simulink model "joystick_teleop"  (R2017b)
settings: Solver=FixedStepDiscrete  StartTime=0.0  StopTime=Inf  FixedStep=0.001  RelTol=1e-3  EnableMultiTasking=on
PostLoadFcn:
  | , if any(exist('dsrtsu_mdlpostloadfcn', 'file') == [2, 3, 6]), try dsrtsu_mdlpostloadfcn('Execute', bdroot); catch fprintf('Error in PostLoadFcn (dsrtsu_mdlpostloadfcn) for model "%s":\n %s\n', bdroot, lasterr); end, end,
libraries: vehicle_data_blocks x9, dbw_interface_blocks x5, adas_kit_info_blocks x2, simulink x2, rtican x1, vehicle_control_blocks x1

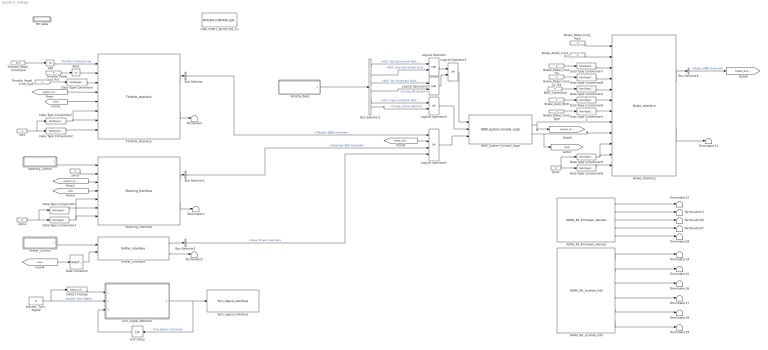
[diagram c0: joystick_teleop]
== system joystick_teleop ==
  ADAS_Kit_Firmware_Version : adas_kit_info_blocks/ADAS_Kit_Firmware_Version
  ADAS_Kit_License_Info : adas_kit_info_blocks/ADAS_Kit_License_Info
  Abs : Abs
  Abs1 : Abs
  BOO_Command : Constant  Value=0
  Brake_Auto_BOO : Constant
  Brake_Interface : dbw_interface_blocks/Brake_Interface
  Brake_Pedal_Cmd_CL_Trq : Constant  Value=0
  Brake_Pedal_Cmd_Pct : Constant  Value=0
  Brake_Pedal_Cmd_Raw : Constant  Value=0
  Brake_Pedal_Cmd_Trq : Constant  Value=0
  Brake_Pedal_Cmd_Type : Constant  Value=3
  Bus Selector : BusSelector  OutputSignals=Throttle_DBW_Override
  Bus Selector1 : BusSelector  OutputSignals=Steering_DBW_Override
  Bus Selector2 : BusSelector  OutputSignals=Gear_Driver_Override
  Bus Selector3 : BusSelector  OutputSignals=ACC_Set_Decrement_Button,ACC_Gap_Decrement_Button,ACC_Set_Increment_Button,Cruise_Off_Button,ACC_Gap_Increment_Button,Cruise_Cancel_Button
  Bus Selector4 : BusSelector  OutputSignals=Brake_DBW_Override
  CAN_TYPE1_SETUP_M1_C1 : rtican/RTICAN CONTROLLER SETUP   Reserved1=[]  Reserved2=[]  Reserved3=[]  Reserved4=[]  AcceptanceMask=[]  ArbitrationField=[]  Parameters=[]  SFcnRTICANSettings=[]  MS_Struct=[]  BoardTypeNo=[]  BoardNo=[]  ChannelNo=[]  DialogFcn=[]  UnitName=[]  Revision=[]  UnitValues=[]  DSProperties=struct('RTI',struct('Version',uint32(12),'BlockType',struct('isSLSource',uint8(0),'isSLSink',uint8(0),'isHWSource',uint8(0),'isHWSink',uint8(0),'isSetup',uint8(1),'isInline',uint8(1),'isNonInline',uint8(0),'isInterrupt',uint8(0),'isChannelwise',uint8(0)),'IOBoardType','RTICAN','UnitType','NON_MESSAGE','Identifier','MASTER','DialogType','ML','BlockSet','RTICAN','SlaveProcessor','CAN'))  RTIBlockInterface=struct('InputPortsWidth',int32(0),'InputPortsActive',0,'OutputPortsWidth',int32(0),'OutputPortsActive',0,'DialogFcn','rtican_master_setup_gui','BlockDisplay',{{['CAN CONTROLLER\n SETUP'],'center'}},'IconTransparency','on','InitLevel',3,'IWork',{{{'',uint32(2)}}},'BlockName',struct('Token',{{'CAN_TYPE','_SETUP_M','_C'}},'BlockParam',{{'BoardTypeNo','BoardNo','ChannelNo'}}),'ParameterTunableNames',{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  RTIBlockParameters=struct('BoardTypeNo',{{1,'OFF',[]}},'BoardNo',{{1,'ON',[1 16]}},'ChannelNo',{{1,'ON',[1 2]}},'AcceptanceMask',{{0,'OFF',[]}},'ArbitrationField',{{0,'OFF',[]}},'Parameters',{{struct('Config',struct('Baudrate',500,'SampleMode',1,'UsedParamSet',1,'validSettings',1,'isBTRvalues',0,'Advanced',struct('Baudrate',{500,500,500},'Frequency',{24000000,36000000,64000000},'Settings',{struct('SMPL',0,'BRP',0,'N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  RTISFcnParameters=struct('SFcnRTICANSettings','struct','SFcnRTICCPSettings','struct','SFcnRTIXCPSettings','struct','AcceptanceMask','int32','ArbitrationField','int32','TLCFileName','char')  RTIBlockParaDefault=struct('BoardTypeNo',4302,'BoardNo',1,'ChannelNo',1,'AcceptanceMask',0,'ArbitrationField',0,'Parameters',struct('Config',struct('Baudrate',500,'SampleMode',1,'UsedParamSet',1,'validSettings',1,'isBTRvalues',0,'Advanced',struct('Frequency',16000000,'BTR0',64,'BTR1',28,'Settings',struct('SMPL',0,'BRP',0,'NBT',16,'TSEG1',12,'TSEG2',1,'SJW',1,'SP',87))),'configType',1,'Options',struct('DataFileSelecte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
  DBW_System_Enable_Logic : vehicle_control_blocks/DBW_System_Enable_Logic
  Data Type Conversion{,2,4,6,11} (5 alike) : DataTypeConversion  OutDataTypeStr=uint8
  Data Type Conversion{1,3,5,9..10} (5 alike) : DataTypeConversion  OutDataTypeStr=boolean
  Data Type Conversion7 : DataTypeConversion  OutDataTypeStr=uint16
  Data Type Conversion8 : DataTypeConversion  OutDataTypeStr=uint16
  Detect Change : simulink/Logic and Bit Operations/Detect Change  vinit=0  OutDataTypeStr=boolean
  Joystick_Turn_Signal : Constant  Value=0
  Logical Operator : Logic  AllPortsSameDT=off  OutDataTypeStr=boolean
  Logical Operator1 : Logic  Operator=OR  Inputs=4  AllPortsSameDT=off  OutDataTypeStr=boolean
  Logical Operator2 : Logic  AllPortsSameDT=off  OutDataTypeStr=boolean
  Logical Operator3 : Logic  Operator=OR  AllPortsSameDT=off  OutDataTypeStr=boolean
  Logical Operator4 : Logic  Operator=OR  AllPortsSameDT=off  OutDataTypeStr=boolean
  RTI Data : Subsystem  Tag=struct('RTIDataServer',struct('RTIDataServerVs','2','RTIModelDescription','struct(''main'',''joystick_teleop'',''sub'','''',''isMp'',0)'))  LoadFcn="if exist('rtidc'), try,  rtidc('DataHostBlockClbLoad', gcbh); catch, disp(['Warning: ''LoadFcn'' for RTI Data block failed: ' lasterr]); end, end,"  mask(RTI_DATA_HOST){}
      mask help: RTI Data Block. This block is used by RTI to store internal model-dependent data. Please keep this block on the root level of the model. Deleting this block will result in data loss. NEVER DELETE OR COPY THIS BLOCK!
  Rate Transition : RateTransition
  Shifter_Control : Subsystem
  Shifter_Interface : dbw_interface_blocks/Shifter_Interface
  Steering_Control : Subsystem
  Steering_Interface : dbw_interface_blocks/Steering_Interface
  Terminator{,1..2,11..19,26..28} (15 alike) : Terminator
  Throttle_Interface : dbw_interface_blocks/Throttle_Interface
  Throttle_Pedal_Cmd_Pct : Constant  Value=0
  Throttle_Pedal_Cmd_Type : Constant  Value=2
  Throttle_Pedal_Command : Constant  Value=0.15
  Turn_Signal_Behavior : MATLAB Function  TreatAsAtomicUnit=on
  Turn_Signal_Interface : dbw_interface_blocks/Turn_Signal_Interface
  Unit Delay : UnitDelay  SampleTime=-1
  Vehicle_Data : Subsystem
  zero{,1..3} (4 alike) : Constant  Value=0
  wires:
  Throttle_Pedal_Command/1 -> Abs/1
  Abs/1 -> Throttle_Interface/1  "Throttle_Command_Sig"
  [system_enable] -> Throttle_Interface/4
  Throttle_Interface/1 -> Bus Selector/1
  Bus Selector/1 -> Logical Operator1/1  "<Throttle_DBW_Override>"
  Steering_Control/1(Steering_Command) -> Steering_Interface/1
  [system_enable] -> Steering_Interface/3
  Steering_Interface/1 -> Bus Selector1/1
  Bus Selector1/1 -> Logical Operator1/3  "<Steering_DBW_Override>"
  Steering_Interface/2 -> Terminator1/1
  Shifter_Control/1(Gear_Command) -> Shifter_Interface/1
  [clear] -> Rate Transition/1
  Rate Transition/1 -> Shifter_Interface/2
  Bus Selector2/1 -> Logical Operator1/4  "<Gear_Driver_Override>"
  Shifter_Interface/1 -> Bus Selector2/1
  Shifter_Interface/2 -> Terminator2/1
  Joystick_Turn_Signal/1 -> Detect Change/1, Turn_Signal_Behavior/2(u)  "Joystick_Turn_Signal"
  Detect Change/1 -> Turn_Signal_Behavior/1(new_u)
  Turn_Signal_Behavior/1(y) -> Turn_Signal_Interface/1, Unit Delay/1  "Turn_Signal_Command"
  Unit Delay/1 -> Turn_Signal_Behavior/3(last_y)
  Vehicle_Data/1(Misc_Report_Bus) -> Bus Selector3/1
  Bus Selector3/1 -> Logical Operator/1  "<ACC_Set_Decrement_Button>"
  Bus Selector3/2 -> Logical Operator/2  "<ACC_Gap_Decrement_Button>"
  Bus Selector3/5 -> Logical Operator4/1  "<ACC_Gap_Increment_Button>"
  [brake_override] -> Logical Operator1/2
  Logical Operator1/1 -> DBW_System_Enable_Logic/3
  DBW_System_Enable_Logic/2 -> [clear], Brake_Interface/9
  Brake_Pedal_Cmd_Raw/1 -> Brake_Interface/1
  Bus Selector4/1 -> [brake_override]  "<Brake_DBW_Override>"
  Bus Selector3/3 -> Logical Operator2/1  "<ACC_Set_Increment_Button>"
  Bus Selector3/4 -> Logical Operator2/2  "<Cruise_Off_Button>"
  Bus Selector3/6 -> Logical Operator4/2  "<Cruise_Cancel_Button>"
  Logical Operator/1 -> Logical Operator3/1
  Logical Operator2/1 -> Logical Operator3/2
  Logical Operator3/1 -> DBW_System_Enable_Logic/1
  Logical Operator4/1 -> DBW_System_Enable_Logic/2
  DBW_System_Enable_Logic/1 -> [system_enable], Brake_Interface/8
  Throttle_Interface/2 -> Terminator/1
  Brake_Interface/2 -> Terminator11/1
  Brake_Interface/1 -> Bus Selector4/1
  ADAS_Kit_License_Info/1 -> Terminator14/1
  ADAS_Kit_License_Info/2 -> Terminator15/1
  ADAS_Kit_License_Info/3 -> Terminator16/1
  ADAS_Kit_License_Info/4 -> Terminator17/1
  ADAS_Kit_License_Info/5 -> Terminator18/1
  ADAS_Kit_License_Info/6 -> Terminator19/1
  [clear] -> Steering_Interface/4
  zero3/1 -> Steering_Interface/2
  ADAS_Kit_Firmware_Version/1 -> Terminator12/1
  ADAS_Kit_Firmware_Version/2 -> Terminator13/1
  ADAS_Kit_Firmware_Version/3 -> Terminator26/1
  ADAS_Kit_Firmware_Version/4 -> Terminator27/1
  ADAS_Kit_Firmware_Version/5 -> Terminator28/1
  zero/1 -> Data Type Conversion2/1, Data Type Conversion1/1
  [clear] -> Throttle_Interface/5
  zero1/1 -> Data Type Conversion6/1, Data Type Conversion5/1
  BOO_Command/1 -> Data Type Conversion10/1
  Brake_Pedal_Cmd_Type/1 -> Data Type Conversion11/1
  Brake_Pedal_Cmd_Trq/1 -> Data Type Conversion7/1
  Brake_Pedal_Cmd_CL_Trq/1 -> Data Type Conversion8/1
  Brake_Pedal_Cmd_Pct/1 -> Brake_Interface/2
  Brake_Auto_BOO/1 -> Data Type Conversion9/1
  Throttle_Pedal_Cmd_Type/1 -> Data Type Conversion/1
  Throttle_Pedal_Cmd_Pct/1 -> Abs1/1
  zero2/1 -> Data Type Conversion4/1, Data Type Conversion3/1
  Data Type Conversion/1 -> Throttle_Interface/3
  Data Type Conversion1/1 -> Throttle_Interface/7, Throttle_Interface/6
  Data Type Conversion2/1 -> Throttle_Interface/8
  Data Type Conversion3/1 -> Steering_Interface/7, Steering_Interface/5
  Data Type Conversion4/1 -> Steering_Interface/6
  Data Type Conversion6/1 -> Brake_Interface/12
  Data Type Conversion5/1 -> Brake_Interface/11, Brake_Interface/10
  Data Type Conversion7/1 -> Brake_Interface/3
  Data Type Conversion8/1 -> Brake_Interface/4
  Data Type Conversion9/1 -> Brake_Interface/6
  Data Type Conversion10/1 -> Brake_Interface/5
  Data Type Conversion11/1 -> Brake_Interface/7
  Abs1/1 -> Throttle_Interface/2

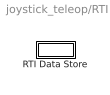
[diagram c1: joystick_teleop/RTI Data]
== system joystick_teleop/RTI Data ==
  RTI Data Store : Subsystem  Tag=struct('private',struct('version',struct('dsVer',uint32(2),'dsVerCreation',uint32(2),'RTI',struct('ver','6.9.1','type','RTI1401')),'access',struct('type','Model','isPerm',1,'created',['03-Jun-2015 12:16:08'],'modified',['23-Jul-2018 12:51:08'],'location','')),'public',struct('main',struct('data',[]),'sub',struct('name',{{'joystick_teleop'}},'data',{{struct('TH',struct('thTaskInfo',struct('taskType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  mask(RTI_DATA_STORE){}
      mask help: RTI Data Store Block. This block is used by RTI to store internal model dependent data. Deleting this block will result in data loss. NEVER DELETE, COPY, OR MODIFY THIS BLOCK!

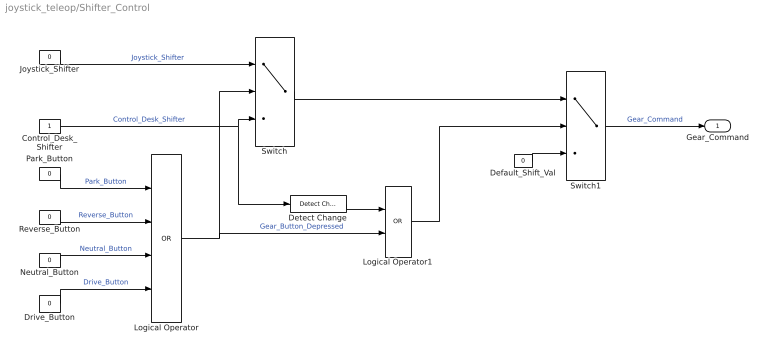
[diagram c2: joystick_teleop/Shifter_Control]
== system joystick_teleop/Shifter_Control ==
  Control_Desk_Shifter : Constant
  Default_Shift_Val : Constant  Value=0
  Detect Change : simulink/Logic and Bit Operations/Detect Change  vinit=0  OutDataTypeStr=boolean
  Drive_Button : Constant  Value=0
  Joystick_Shifter : Constant  Value=0
  Logical Operator : Logic  Operator=OR  Inputs=4  AllPortsSameDT=off  OutDataTypeStr=boolean
  Logical Operator1 : Logic  Operator=OR  AllPortsSameDT=off  OutDataTypeStr=boolean
  Neutral_Button : Constant  Value=0
  Park_Button : Constant  Value=0
  Reverse_Button : Constant  Value=0
  Switch : Switch  Criteria=u2 ~= 0
  Switch1 : Switch  Criteria=u2 ~= 0
  Gear_Command : Outport
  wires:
  Park_Button/1 -> Logical Operator/1  "Park_Button"
  Reverse_Button/1 -> Logical Operator/2  "Reverse_Button"
  Neutral_Button/1 -> Logical Operator/3  "Neutral_Button"
  Drive_Button/1 -> Logical Operator/4  "Drive_Button"
  Logical Operator/1 -> Switch/2, Logical Operator1/2  "Gear_Button_Depressed"
  Control_Desk_Shifter/1 -> Detect Change/1, Switch/3  "Control_Desk_Shifter"
  Joystick_Shifter/1 -> Switch/1  "Joystick_Shifter"
  Detect Change/1 -> Logical Operator1/1
  Switch1/1 -> Gear_Command/1  "Gear_Command"
  Switch/1 -> Switch1/1
  Default_Shift_Val/1 -> Switch1/3
  Logical Operator1/1 -> Switch1/2

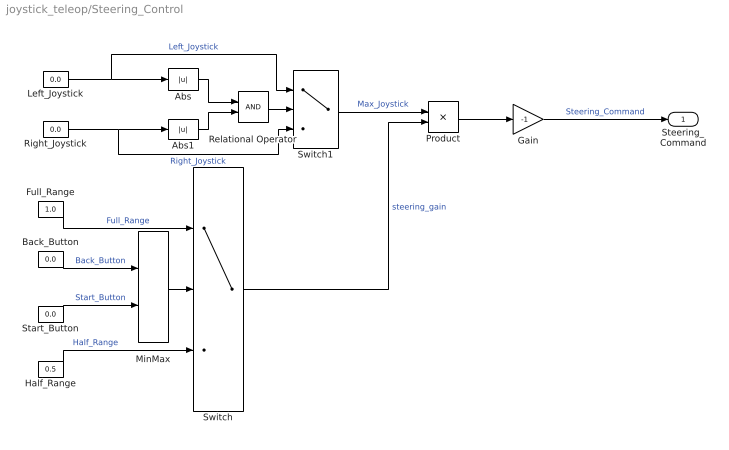
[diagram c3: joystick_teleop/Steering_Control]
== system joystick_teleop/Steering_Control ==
  Abs : Abs
  Abs1 : Abs
  Back_Button : Constant  Value=0.0
  Full_Range : Constant  Value=1.0
  Gain : Gain  Gain=-1
  Half_Range : Constant  Value=0.5
  Left_Joystick : Constant  Value=0.0
  MinMax : MinMax  Function=max  Inputs=2
  Product : Product
  Relational Operator : RelationalOperator  OutDataTypeStr=boolean
  Right_Joystick : Constant  Value=0.0
  Start_Button : Constant  Value=0.0
  Switch : Switch  Criteria=u2 ~= 0
  Switch1 : Switch  Criteria=u2 ~= 0
  Steering_Command : Outport
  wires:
  Back_Button/1 -> MinMax/1  "Back_Button"
  Start_Button/1 -> MinMax/2  "Start_Button"
  MinMax/1 -> Switch/2
  Full_Range/1 -> Switch/1  "Full_Range"
  Half_Range/1 -> Switch/3  "Half_Range"
  Left_Joystick/1 -> Abs/1, Switch1/1  "Left_Joystick"
  Right_Joystick/1 -> Switch1/3, Abs1/1  "Right_Joystick"
  Abs/1 -> Relational Operator/1
  Abs1/1 -> Relational Operator/2
  Relational Operator/1 -> Switch1/2
  Switch1/1 -> Product/1  "Max_Joystick"
  Switch/1 -> Product/2  "steering_gain"
  Product/1 -> Gain/1
  Gain/1 -> Steering_Command/1  "Steering_Command"

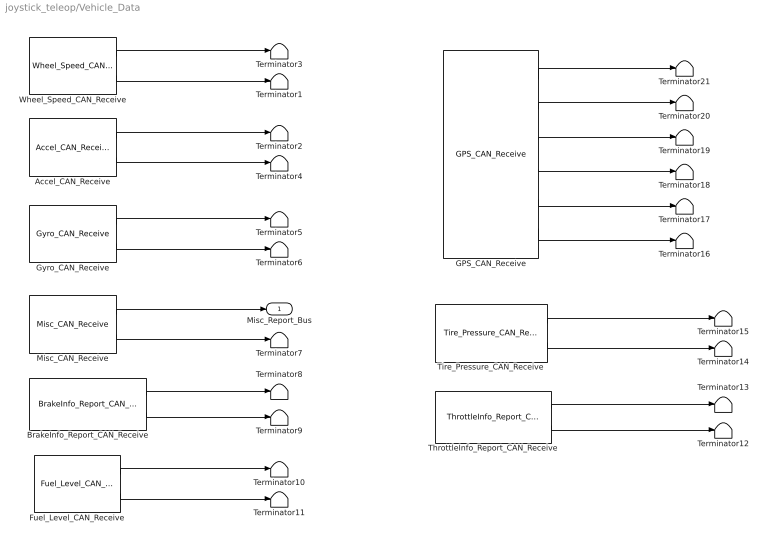
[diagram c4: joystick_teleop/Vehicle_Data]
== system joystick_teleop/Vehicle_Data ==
  Accel_CAN_Receive : vehicle_data_blocks/Accel_CAN_Receive
  BrakeInfo_Report_CAN_Receive : vehicle_data_blocks/BrakeInfo_Report_CAN_Receive
  Fuel_Level_CAN_Receive : vehicle_data_blocks/Fuel_Level_CAN_Receive
  GPS_CAN_Receive : vehicle_data_blocks/GPS_CAN_Receive
  Gyro_CAN_Receive : vehicle_data_blocks/Gyro_CAN_Receive
  Misc_CAN_Receive : vehicle_data_blocks/Misc_CAN_Receive
  Terminator{1..21} (21 alike) : Terminator
  ThrottleInfo_Report_CAN_Receive : vehicle_data_blocks/ThrottleInfo_Report_CAN_Receive
  Tire_Pressure_CAN_Receive : vehicle_data_blocks/Tire_Pressure_CAN_Receive
  Wheel_Speed_CAN_Receive : vehicle_data_blocks/Wheel_Speed_CAN_Receive
  Misc_Report_Bus : Outport
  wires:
  Wheel_Speed_CAN_Receive/1 -> Terminator3/1
  Wheel_Speed_CAN_Receive/2 -> Terminator1/1
  Accel_CAN_Receive/1 -> Terminator2/1
  Accel_CAN_Receive/2 -> Terminator4/1
  Gyro_CAN_Receive/1 -> Terminator5/1
  Gyro_CAN_Receive/2 -> Terminator6/1
  Misc_CAN_Receive/1 -> Misc_Report_Bus/1
  Misc_CAN_Receive/2 -> Terminator7/1
  BrakeInfo_Report_CAN_Receive/1 -> Terminator8/1
  BrakeInfo_Report_CAN_Receive/2 -> Terminator9/1
  Fuel_Level_CAN_Receive/1 -> Terminator10/1
  Fuel_Level_CAN_Receive/2 -> Terminator11/1
  Tire_Pressure_CAN_Receive/1 -> Terminator15/1
  Tire_Pressure_CAN_Receive/2 -> Terminator14/1
  GPS_CAN_Receive/2 -> Terminator20/1
  GPS_CAN_Receive/6 -> Terminator16/1
  GPS_CAN_Receive/3 -> Terminator19/1
  GPS_CAN_Receive/1 -> Terminator21/1
  GPS_CAN_Receive/4 -> Terminator18/1
  GPS_CAN_Receive/5 -> Terminator17/1
  ThrottleInfo_Report_CAN_Receive/2 -> Terminator12/1
  ThrottleInfo_Report_CAN_Receive/1 -> Terminator13/1

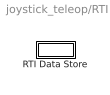
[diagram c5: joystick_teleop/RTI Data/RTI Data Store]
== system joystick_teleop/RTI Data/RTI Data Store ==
  RTI Data Store : Subsystem  mask(RTI_DATA_STORE){}
      mask help: RTI Data Store Block. This block is used by RTI to store internal model dependent data. Deleting this block will result in data loss. NEVER DELETE, COPY, OR MODIFY THIS BLOCK!

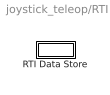
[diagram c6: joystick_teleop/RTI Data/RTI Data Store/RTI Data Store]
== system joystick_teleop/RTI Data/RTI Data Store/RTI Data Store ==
  RTI Data Store : Subsystem  mask(RTI_DATA_STORE){}
      mask help: RTI Data Store Block. This block is used by RTI to store internal model dependent data. Deleting this block will result in data loss. NEVER DELETE, COPY, OR MODIFY THIS BLOCK!

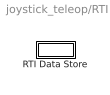
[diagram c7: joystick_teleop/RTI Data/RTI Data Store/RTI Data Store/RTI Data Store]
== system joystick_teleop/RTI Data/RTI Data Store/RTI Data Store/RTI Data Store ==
  RTI Data Store : Subsystem  mask(RTI_DATA_STORE){}
      mask help: RTI Data Store Block. This block is used by RTI to store internal model dependent data. Deleting this block will result in data loss. NEVER DELETE, COPY, OR MODIFY THIS BLOCK!

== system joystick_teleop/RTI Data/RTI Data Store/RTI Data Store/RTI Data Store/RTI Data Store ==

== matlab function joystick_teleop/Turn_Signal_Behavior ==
%% Function Name: Turn_Signal_Fcn
% 
% Description: Implements logic to control the turn signals using the D-pad
%   on the joystick.
%
% Assumptions: None
%
% Inputs:                                                   Size    
%   Flag indicating that the joystick signal has changed    1x1        
%   Current value of the joystick D-pad signal              1x1
%   Previously generated turn signal commmand               1x1
%
% Outputs:                                                  Size
%   Actual turn signal command                              1x1
%
% $Revision: 1.0$
% $Author: Micho Radovnikovich$
% $Date: August 3, 2015$
%
%-----------------------------------------

function y = Turn_Signal_Fcn(new_u, u, last_y)

NONE = 0;
LEFT = 1;
RIGHT = 2;

y = last_y;

if new_u > 0
    if last_y == NONE
        if u ~= NONE
            y = u;
        end
    elseif last_y == RIGHT
        if u == RIGHT
            y = NONE;
        elseif u == LEFT
            y = LEFT;
        end
    else
        if u == LEFT
            y = NONE;
        elseif u == RIGHT
            y = RIGHT;
        end
    end
end
